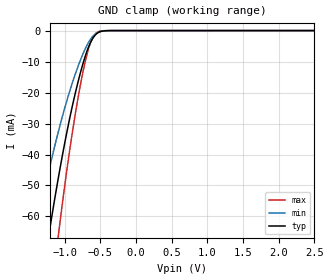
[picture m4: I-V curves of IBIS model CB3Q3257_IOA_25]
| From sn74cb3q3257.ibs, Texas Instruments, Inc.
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[Model]   CB3Q3257_IOA_25
Model_type  Terminator
| variable   typ   min   max
C_comp   5.28pF   3.41pF   9.70pF
| C_tri-state   5.28pF   3.41pF   9.70pF
[Temperature Range]   40   100   -40
| Ambient temperature   25   85   -40
[Voltage range]   2.5   2.3   2.7
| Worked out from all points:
|   GND clamp passes 1 mA (typ) near -0.55 V on its own axis
[GND Clamp]
| CB3Q3257_IOA_25
|   Voltage   I(typ)   I(min)   I(max)
-5.5V     -936.3mA   -734.9mA   -1.142A
-1.4V     -93.35mA   -64.43mA   -129.4mA
-1.21V    -64.47mA   -44.26mA   -89.88mA
-1.09V    -47.94mA   -32.91mA   -66.66mA
-1.07V    -45.34mA   -31.14mA   -62.96mA
-930mV    -28.56mA   -19.72mA   -38.92mA
-850mV    -20.26mA   -14.06mA   -27mA
-760mV    -12.12mA   -8.508mA   -15.39mA
-645mV    -4.293mA   -3.108mA   -4.499mA
-545mV    -907uA     -714.8uA   -587.9uA
-345mV    -5.71uA    -8.569uA   -618.3nA
2.5V      147.2pA    716.2pA    14.5pA
